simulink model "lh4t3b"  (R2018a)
settings: Solver=ode45  StartTime=0.0  StopTime=0.001  RelTol=1e-3  AbsTol=1e-6
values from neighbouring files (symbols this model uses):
  a = 0.01    [lh4t3_m.m]
  K = hairio    (= 1)    [lh4t3_m.m]
  x_1_0 = 5.0    (= 5)    [lh4t3_m.m]
  x_2_0 = 0.0    (= 0)    [lh4t3_m.m]
libraries: simulink x1

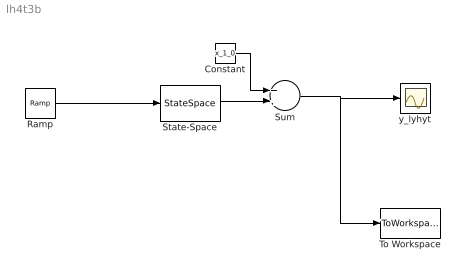
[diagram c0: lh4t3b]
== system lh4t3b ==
  Constant : Constant  Value=x_1_0
  Ramp : simulink/Sources/Ramp  slope=a  start=0  InitialOutput=K
  State-Space : StateSpace  A=-1000  B=1000  D=0  InitialCondition=x_2_0
  Sum : Sum
  To Workspace : ToWorkspace  VariableName=y_lyhyt  SampleTime=-1
  y_lyhyt : Scope
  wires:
  Sum/1 -> y_lyhyt/1, To Workspace/1
  State-Space/1 -> Sum/2
  Constant/1 -> Sum/1
  Ramp/1 -> State-Space/1
